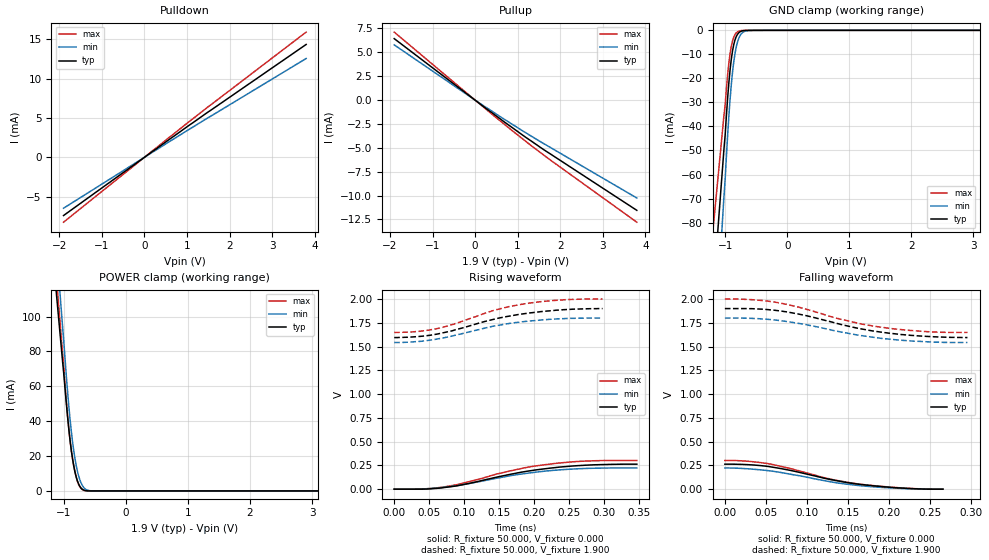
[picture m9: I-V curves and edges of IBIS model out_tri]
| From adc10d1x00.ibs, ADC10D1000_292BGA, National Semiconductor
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[Model]   out_tri
Model_type 3-state
Vref=0.000E+00
Rref=1.000E+06
Cref=0.000E+00
Vmeas=9.500E-01
C_comp   8.33E-13   8.33E-13   8.33E-13
[Voltage Range]   1.900E+00   1.800E+00   2.000E+00
[POWER Clamp Reference]   1.900E+00   1.800E+00   2.000E+00
[GND Clamp Reference]   0.000E+00   0.000E+00   0.000E+00
[Pullup Reference]   1.900E+00   1.800E+00   2.000E+00
[Pulldown Reference]   0.000E+00   0.000E+00   0.000E+00
[Temperature Range]   25   85   -40
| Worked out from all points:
|   slope of the pulldown table from 0 to 0.285 V, typ, clamps not added: 258 ohm
|   slope of the pullup table from 0 to 0.285 V, typ, clamps not added: 295 ohm
|   GND clamp passes 1 mA (typ) near -0.78 V on its own axis
|   POWER clamp passes 1 mA (typ) near -0.70 V on its own axis
|   rising waveform, R_fixture 50.000, V_fixture 0.000: 20-80 % time 109ps typ, 106ps min, 103ps max; typ from 0 V to 0.263 V
|   falling waveform, R_fixture 50.000, V_fixture 0.000: 20-80 % time 90.6ps typ, 90.4ps min, 91.2ps max; typ from 0.263 V to 0 V
|   rising waveform, R_fixture 50.000, V_fixture 1.900: 20-80 % time 102ps typ, 97.3ps min, 93.5ps max; typ from 1.59 V to 1.9 V
|   falling waveform, R_fixture 50.000, V_fixture 1.900: 20-80 % time 95.7ps typ, 97.5ps min, 96.6ps max; typ from 1.9 V to 1.59 V
[GND Clamp]
-1.9V     -351.8mA   -438.2mA   -273mA
-1.02V    -49.71mA   -69.63mA   -35.61mA
-1V       -43.68mA   -61.97mA   -31.07mA
-960mV    -28.23mA   -43.73mA   -18.53mA
-940mV    -21.75mA   -35.68mA   -13.54mA
-900mV    -11.87mA   -22.35mA   -6.507mA
-860mV    -5.808mA   -12.89mA   -2.738mA
-840mV    -3.899mA   -9.466mA   -1.694mA
-800mV    -1.624mA   -4.773mA   -596uA
-720mV    -214.1uA   -947.4uA   -60.72uA
-580mV    -22uA      -46.88uA   -22.11uA
3.8V      0A         0A         0A
[Power Clamp]
-1.9V     417.6mA    498.1mA    464.3mA
-1.02V    74.24mA    94.17mA    78.84mA
-940mV    42.75mA    57.12mA    43.38mA
-900mV    29.28mA    41.21mA    29.02mA
-880mV    23.56mA    34.38mA    23.27mA
-840mV    14.4mA     23.01mA    14.35mA
-800mV    7.963mA    14.46mA    7.843mA
-760mV    3.863mA    8.386mA    3.603mA
-700mV    899.3uA    3.018mA    706.3uA
-640mV    121.5uA    763.3uA    84.45uA
-520mV    0A         0A         0A
3.8V      0A         0A         0A
[Pullup]
-1.9V     6.437mA    5.784mA    7.122mA
220mV     -746.8uA   -656.2uA   -817.4uA
1.2V      -3.926mA   -3.441mA   -4.351mA
1.76V     -5.612mA   -4.936mA   -6.246mA
3.8V      -11.54mA   -10.25mA   -12.78mA
[Pulldown]
-1.9V     -7.385mA   -6.457mA   -8.23mA
1.04V     4.03mA     3.523mA    4.492mA
1.48V     5.695mA    4.979mA    6.346mA
3.8V      14.33mA    12.55mA    15.9mA
[Rising Waveform]
R_fixture = 50.000
V_fixture = 0.000
V_fixture_min = 0.000
V_fixture_max = 0.000
|  time   V(typ)   V(min)   V(max)
0s        0V         0V         0V
41ps      189.4uV    2.886mV    2.164mV
73ps      18.46mV    21.11mV    25.23mV
93ps      40.12mV    40.27mV    52.45mV
147ps     127.2mV    115.6mV    159.6mV
183ps     180.1mV    160mV      219.2mV
199ps     198.5mV    175.8mV    240.8mV
228ps     225.1mV    197.9mV    268.8mV
273ps     251.7mV    217.6mV    295.4mV
347ps     262.9mV    223.2mV    302.1mV
[Falling Waveform]
R_fixture = 50.000
V_fixture = 0.000
V_fixture_min = 0.000
V_fixture_max = 0.000
|  time   V(typ)   V(min)   V(max)
0s        262.9mV    223.2mV    302.1mV
25ps      259mV      215.9mV    295.6mV
54ps      237.3mV    193.7mV    266.5mV
82ps      193.7mV    154mV      212.7mV
131ps     97.8mV     74.58mV    101.4mV
165ps     50.03mV    36.77mV    52.51mV
191ps     27.58mV    18.61mV    29.35mV
218ps     10.23mV    6.538mV    11.67mV
244ps     605.2uV    341.6uV    2.208mV
266ps     0V         0V         0V
[Rising Waveform]
R_fixture = 50.000
V_fixture = 1.900
V_fixture_min = 1.800
V_fixture_max = 2.000
|  time   V(typ)   V(min)   V(max)
0s        1.595V     1.543V     1.649V
37ps      1.607V     1.555V     1.661V
68ps      1.642V     1.588V     1.7V
88ps      1.678V     1.621V     1.743V
144ps     1.79V      1.718V     1.884V
165ps     1.821V     1.744V     1.922V
182ps     1.842V     1.76V      1.945V
210ps     1.868V     1.78V      1.973V
248ps     1.89V      1.796V     1.995V
298ps     1.9V       1.8V       2V
[Falling Waveform]
R_fixture = 50.000
V_fixture = 1.900
V_fixture_min = 1.800
V_fixture_max = 2.000
|  time   V(typ)   V(min)   V(max)
0s        1.9V       1.8V       2V
39ps      1.897V     1.794V     1.99V
57ps      1.886V     1.783V     1.973V
75ps      1.866V     1.764V     1.945V
99ps      1.826V     1.731V     1.893V
137ps     1.743V     1.661V     1.797V
167ps     1.685V     1.615V     1.737V
193ps     1.649V     1.584V     1.701V
246ps     1.607V     1.551V     1.657V
296ps     1.595V     1.543V     1.649V
[Ramp]
dV/dt_r   1.5053E-01/1.0953E-10   1.2764E-01/1.0569E-10   1.7039E-01/1.0278E-10
dV/dt_f   1.8285E-01/9.5312E-11   1.5447E-01/9.7437E-11   2.1040E-01/9.5937E-11
R_load = 50
